PROGRAM Prg_Vision
VAR
	aColorRed 			: TcVnVector4_LREAL := [255, 0, 0];
	aColorGreen 		: TcVnVector4_LREAL := [0, 255, 0];
	aColorBlue 			: TcVnVector4_LREAL := [0, 0, 255];
	
	FBProfiler			: Profiler;
		
	hr  				: HRESULT;
    fbCamera			: FB_VN_SimpleCameraControl;
    eState				: ETcVnCameraState;
     
	udWidth				: UDINT;
	udHeight			: UDINT;	
    ipImageIn 			: ITcVnImage;
    ipImageInDisp 		: ITcVnDisplayableImage;
	
	
	ipImageRes 			: ITcVnImage;
	ipImageResDisp 		: ITcVnDisplayableImage;

	stDrawRoi			: TcVnRectangle_UDINT := (nX := 900, nY := 850, nWidth := 1000, nHeight := 1000);	
	stRoi				: TcVnRectangle_UDINT := (nX := 900, nY := 850, nWidth := 1000, nHeight := 1000);
	ipContourList1		: ITcVnContainer;
	
	ipImageRegion 		: ITcVnImage;
    ipImageRegionDisp	: ITcVnDisplayableImage;
	
	aOffset1			: TcVnPoint;
	nNumberOfElements	: ULINT;
	iRef1				: ULINT;
	fArea1				: LREAL;
	ipContour1			: ITcVnContainer;
	iDetectNum1			: INT;
	fCircularity		:LREAL;
	fAngle_M1			: LREAL;	
	sAngle_M1			: STRING(20);	
	stRectangle			: TcVnRotatedRectangle;		
	
	ipStructimage 		: ITcVnImage;
	certerofmass		: TcVnPoint2_LREAL;
	aEndPoint			: TcVnPoint2_REAL;
	
	eDirection			: ETcVnEdgeDirection := TCVN_ED_DARK_TO_LIGHT;	
	fMinStrength		: REAL := 50;
	nSearchLines		: UDINT := 101;
	fSearchLineDist		: REAL := 3;
	nMaxThickness		: UDINT := 1;
	nSubpixIter			: UDINT := 10;
	eAlgorithm			: ETcVnEdgeDetectionAlgorithm := TCVN_EDA_INTERPOLATION;
	fAvgStrength		: REAL;
	ipEdgePoints		: ITcVnContainer;	
	aLine				: TcVnVector4_LREAL;
	aStartPoint			: TcVnPoint2_REAL;
	fAngle_M2			: LREAL;
	sAngle_M2			: STRING(20);
	
	fHideth				: REAL;
	circleofMass		: TcVnPoint2_LREAL;
	L					: LREAL;
	X1					: LREAL;
	Y1					: LREAL;
	L1					: REAL;
	
	lasttime			: LREAL;
	maxtime				: LREAL;
	averagetime			: REAL;
	mintime				: REAL;
	bFindAngle_M1Temp   : BOOL;
	
	// 形态学开闭算法切换
	eOperator			: ETcVnMorphologicalOperator := ETcVnMorphologicalOperator.TCVN_MO_CLOSING;
	// 形态学卷积核
	udStructElement		: UDINT := 10;
	// 形态学启用		
	bmorphology			: BOOL;
	// 模式切换
	bModeSwitch			: BOOL;
	// OK、NG信号
	bFindAngle_M1		: BOOL;
	bFindAngle_M2		: BOOL;
END_VAR

eState := fbCamera.GetState();
CASE eState OF
TCVN_CS_INITIAL,TCVN_CS_OPENING,TCVN_CS_OPENED,TCVN_CS_STARTACQUISITION:
    hr := fbCamera.StartAcquisition();
TCVN_CS_ACQUIRING:
    hr := fbCamera.GetCurrentImage(ipImageIn);
    IF SUCCEEDED(hr) AND ipImageIn <> 0 THEN
		FBProfiler(START:=FALSE , RESET:=TRUE , BUSY=> , DATA=> );
		FBProfiler(START:=TRUE , RESET:=FALSE , BUSY=> , DATA=> );	
		
		hr := F_VN_GetImageWidth(ipImage:=ipImageIn , nWidth:=udWidth , hr );
		hr := F_VN_GetImageHeight(ipImage:=ipImageIn , nHeight:=udHeight , hr );
		// 图像色彩转换
		hr := F_VN_ConvertColorSpace(ipImageIn,ipImageRes,TCVN_CST_GRAY_TO_RGB, hr );
		
		A10_MakeRegion();
		//模式切换
		IF NOT bModeSwitch THEN
			A20_FindContours();
		ELSE
			A20_FindContours();
			A30_LocateEdge();
		END_IF
		// 窗口输出
		hr := F_VN_TransformIntoDisplayableImage(ipImageIn,ipImageInDisp, S_OK );
		hr := F_VN_TransformIntoDisplayableImage(ipImageRegion,ipImageRegionDisp, S_OK );	
		hr := F_VN_TransformIntoDisplayableImage(ipImageRes,ipImageResDisp, S_OK );	
		
		FBProfiler(START:=FALSE , RESET:=FALSE , BUSY=> , DATA=> );
    END_IF
TCVN_CS_ERROR:
    hr := fbCamera.Reset();
END_CASE

// 执行时间统计
lasttime:=   (DWORD_TO_REAL(FBprofiler.DATA.LastExecTime))/1000;
maxtime:=  (DWORD_TO_REAL( FBprofiler.DATA.MaxExecTime))/1000;
mintime:= (DWORD_TO_REAL( FBprofiler.DATA.MinExecTime))/1000;
averagetime:=(DWORD_TO_REAL( FBprofiler.DATA.AverageExecTime))/1000;

ACTION A10_MakeRegion:
// 检测区域(ROI)选定
hr := F_VN_CopyImageRegion(
			ipSrcImage:=ipImageIn , 
			nX:=stRoi.nX , 
			nY:=stRoi.nY , 
			nWidth:=stRoi.nWidth , 
			nHeight:=stRoi.nHeight , 
			ipDestImage:=ipImageRegion , 
			hrPrev:=hr );

// C#调试界面实现鼠标选定框, 并由C#传递给 F_VN_CopyImageRegion 进行动态区域选定
IF stDrawRoi.nWidth <= udWidth AND stDrawRoi.nHeight <= udHeight THEN
	hr := F_VN_DrawRectangle_TcVnRectangle_UDINT(stDrawRoi,ipImageRes,aColorRed,5,hr);		
END_IF
		
// 绘制检测区域(ROI)
hr := F_VN_DrawRectangle_TcVnRectangle_UDINT(stRoi,ipImageRes,aColorBlue,5,hr);

// 二值化
hr := F_VN_Threshold(
			ipSrcImage:=ipImageRegion , 
			ipDestImage:=ipImageRegion , 
			fThreshold:=0 , 
			fMaxValue:=255 , 
			eThresholdType:=TCVN_TT_OTSU_BINARY_INV , 
			hrPrev:=hr );
			
// 形态学处理（腐蚀、膨胀）
IF bmorphology THEN	
hr := F_VN_CreateStructuringElement(ipStructimage ,TCVN_SES_RECTANGLE ,udStructElement ,udStructElement ,hr );
hr := F_VN_MorphologicalOperator( ipImageRegion,ipImageRegion ,eOperator ,ipStructimage ,hr );	
END_IF
END_ACTION

ACTION A20_FindContours:
aOffset1[0] := 	stRoi.nX;
aOffset1[1] := 	stRoi.nY;	
// 获取轮廓列表
hr := F_VN_FindContoursExp(
			ipSrcImage:=ipImageRegion , 
			ipContours:=ipContourList1 , 
			eRetrievalMode:=TCVN_CRM_LIST , 
			eApproximationMethod:=TCVN_CAM_SIMPLE , 
			aOffset:=aOffset1 , 
			hrPrev:=hr );
			
bFindAngle_M1Temp :=FALSE;
// 获取轮廓数量
hr := F_VN_GetNumberOfElements(ipContourList1 , nNumberOfElements , hr );
iDetectNum1:=0;
IF nNumberOfElements>=1 THEN
	FOR iRef1:=0 TO (nNumberOfElements-1) DO
		// 依次获取容器中所有识别的轮廓
		hr := F_VN_GetAt_ITcVnContainer(ipContourList1 ,ipContour1 ,iRef1 , hr );
		// 依次获取容器中所有识别的轮廓面积
		hr := F_VN_ContourArea(ipContour1 , fArea1 , hr );
		IF fArea1>10000 THEN
			IF fArea1>300000 AND fArea1<800000 AND bModeSwitch THEN
				// 获取轮廓质心
				F_VN_ContourCenterOfMass(ipContour1,circleofmass,hr);
				// 绘制轮廓
				hr := F_VN_DrawContours(ipContour1, -1, ipImageRes, aColorGreen, 5, hr);
				// 绘制质心坐标
				hr := F_VN_DrawPointExp(LREAL_TO_UDINT(circleofmass[0]), LREAL_TO_UDINT(circleofmass[1]), ipImageRes, TCVN_DS_X, aColorBlue,5,5,TCVN_LT_4_CONNECTED, hr);
			END_IF	
			// 获取弧度
			hr := F_VN_ContourCircularity(ipContour1,fCircularity,hr);
			// 通过弧度排除中间的圆
			IF(fCircularity< 0.6) THEN
				iDetectNum1:=iDetectNum1+1;
				IF(iDetectNum1 = 1) THEN
					// 获取轮廓质心
					hr := F_VN_ContourCenterOfMass(ipContour1,certerofmass,hr);
					// 提取外接矩形关键特征
					hr := F_VN_EnclosingRectangle(ipContour1,stRectangle,hr);	
					// 绘制外接矩形轮廓
					hr := F_VN_DrawRotatedRectangle(stRectangle,  ipImageRes, aColorGreen, 5, hr);
					IF SUCCEEDED(hr)  THEN
						bFindAngle_M1Temp :=TRUE;
					END_IF
					// 提取矩形宽度、角度特征
					fHideth := stRectangle.stSize.fHeight;
					IF NOT bModeSwitch THEN
						fAngle_M1 := stRectangle.fAngle;
						IF stRectangle.fAngle >90 THEN
							fAngle_M1 := 180-stRectangle.fAngle;
						END_IF
						sAngle_M1:=CONCAT('Mode1 Angle: ' , TO_STRING(fAngle_M1));
						// 绘制模式一的角度结果
						hr := F_VN_PutTextExp(sAngle_M1, ipImageRes, 25, 300, ETcVnFontType.TCVN_FT_HERSHEY_PLAIN,6,aColorGreen,5,TCVN_LT_4_CONNECTED, FALSE, hr);
					END_IF
				END_IF	
			END_IF
		END_IF
	END_FOR
END_IF
bFindAngle_M1 := bFindAngle_M1Temp;
// 内存释放，防止溢出
FW_SafeRelease(ADR(ipContourList1) );
FW_SafeRelease(ADR(ipContour1) );
END_ACTION

ACTION A30_LocateEdge:
// 质心获取起点
aStartPoint[0]:=certerofmass[0];
aStartPoint[1]:=certerofmass[1];

// 等比算法动态获取终点
X1:=circleofmass[0]-certerofmass[0];
Y1:=circleofmass[1]-certerofmass[1];
L:=SQRT(X1*X1+Y1*Y1);
L1:=fHideth;
aEndpoint[0]:=certerofmass[0]-L1*(circleofmass[0]-certerofmass[0])/L;
aEndpoint[1]:=certerofmass[1]-L1*(circleofmass[1]-certerofmass[1])/L;

// 绘制起点与重点坐标
hr := F_VN_DrawPointExp(REAL_TO_UDINT(aStartPoint[0]), REAL_TO_UDINT(aStartPoint[1]), ipImageRes, TCVN_DS_X, aColorRed,5,5,TCVN_LT_4_CONNECTED, hr);
hr := F_VN_DrawPointExp(REAL_TO_UDINT(aEndPoint[0]), REAL_TO_UDINT(aEndPoint[1]), ipImageRes, TCVN_DS_X, aColorRed,5,5,TCVN_LT_4_CONNECTED, hr);

// 寻找起点与终点间的边界
hr := F_VN_LocateEdgeExp(
						ipSrcImage				:= ipImageIn, 
						ipEdgePoints			:= ipEdgePoints, 
						aStartPoint				:= aStartPoint, 
						aEndPoint				:= aEndPoint, 
						eEdgeDirection			:= eDirection, 
						fMinStrength			:= fMinStrength, 
						nSearchLines			:= nSearchLines,
						fSearchLineDist			:= fSearchLineDist, 
						nMaxThickness			:= nMaxThickness, 
						nSubpixelsIterations	:= nSubpixIter, 
						fApproxPrecision		:= 0.0001, 
						eAlgorithm				:= eAlgorithm, 
						hrPrev					:= hr, 
						fAvgStrength			=> fAvgStrength);

// 拟合直线
hr := F_VN_FitLine(ipEdgePoints, aLine, hr);
IF SUCCEEDED(hr) THEN
	bFindAngle_M2 := TRUE;
ELSE
	bFindAngle_M2 := FALSE;
END_IF
// 绘制直线
hr := F_VN_DrawLine_TcVnVector4_LREAL(aLine, ipImageRes, aColorRed, 5, hr);
// 绘制边界点
hr := F_VN_DrawPointsExp(ipEdgePoints, ipImageRes, TCVN_DS_PLUS, aColorBlue, 1, 1, TCVN_LT_8_CONNECTED, hr);	

// 算角度
fAngle_M2:=ABS(ATAN(aLine[1]/aLine[0])/PI*180);
sAngle_M2:=CONCAT('Mode2 Angle: ' , TO_STRING(fAngle_M2));
// 绘制模式二的角度结果
IF bModeSwitch THEN
	hr := F_VN_PutTextExp(sAngle_M2, ipImageRes, 25, 450, ETcVnFontType.TCVN_FT_HERSHEY_PLAIN,6,aColorRed,5, TCVN_LT_4_CONNECTED, FALSE, hr);
END_IF

// 内存释放，防止溢出
FW_SafeRelease(ADR(ipContourList1) );
FW_SafeRelease(ADR(ipContour1) );
END_ACTION

END_PROGRAM
